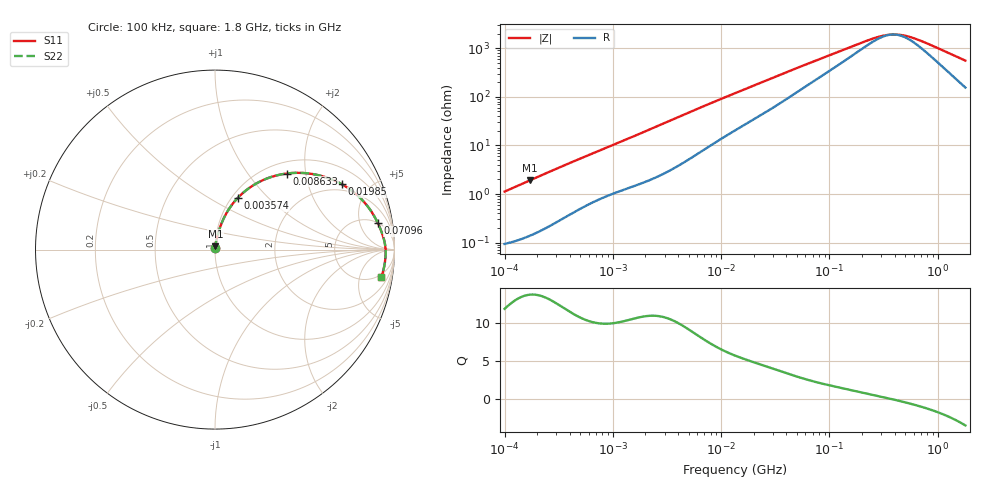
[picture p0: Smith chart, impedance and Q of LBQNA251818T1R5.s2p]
! LBQNA251818T1R5  S-PARAMETER MODEL  ( General Type )
! Model Generated by TAIYO YUDEN Corporation (http://www.ty-top.com)
! Version 1.0
! TAIYO YUDEN Control No. 191025NI43SB-FBB
! Copyright(c) 2019 TAIYO YUDEN CO.,LTD. All Rights Reserved.
! Product Description (link to TY-COMPAS)
! https://ds.yuden.co.jp/TYCOMPAS/or/detail?pn=LBQNA251818T1R5M&u=M
! Products Name : Inductors
! Characteristics :
!  Inductance : 1.5 uH , SRF(min) : 80 MHz , DC Resistance(max) : 0.091 Ohm
!  Rated Current : Saturation :650 mA , Temp Rise : 1100 mA (20 degC)
!  Case Size : 2.5 x 1.8 / 0.098 x 0.071 [mm/inch] , Thickness : 1.8 / 0.071 [mm/inch]
!  (Conditions: Temperature = 25 degC , DC Bias Current/Voltage = 0A / 0V)
! External Node Assignments :
!  1  o---GGG---o  2
! GND o---------o GND
! Frequency Range : 0.1MHz  -  1800MHz  [ 402 STEP ]
# MHz S RI R 50
! Freq[MHz].  S11 Real  S11 Imag  S21 Real  S21 Imag  S12 Real  S12 Imag  S22 Real  S22 Imag
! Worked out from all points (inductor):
!   401 points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, 100 kHz to 1.8 GHz, reference 50 ohm
!   read as one part in series: L = 1.78 uH near 105 kHz
!   highest Q = 13.8 at 171.4 kHz (marker M1), where L = 1.78 uH
!   self-resonance near 382.3 MHz
!   S11 on the Smith chart (normalised r, x): 100 kHz: 1.00, +0.02; 3.574 MHz: 1.07, +0.68; 8.633 MHz: 1.22, +1.57; 19.85 MHz: 1.68, +3.32; 70.96 MHz: 5, +10; 1.8 GHz: 4, -11
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0.1  0.00107 0.0112  0.9989 -0.0112  0.9989 -0.0112  0.00107 0.0112
0.171412  0.00175 0.0191  0.9982 -0.0191  0.9982 -0.0191  0.00175 0.0191
0.516129  0.00813 0.0544  0.9919 -0.0544  0.9919 -0.0544  0.00813 0.0544
1.246616  0.0268 0.1198  0.9732 -0.1198  0.9732 -0.1198  0.0268 0.1198
2.66389  0.0809 0.2308  0.9191 -0.2308  0.9191 -0.2308  0.0809 0.2308
3.574164  0.1272 0.2885  0.8728 -0.2885  0.8728 -0.2885  0.1272 0.2885
5.420303  0.2319 0.3694  0.7681 -0.3694  0.7681 -0.3694  0.2319 0.3694
8.632747  0.3996 0.424  0.6004 -0.424  0.6004 -0.424  0.3996 0.424
13.41641  0.5727 0.4153  0.4273 -0.4153  0.4273 -0.4153  0.5727 0.4153
19.85396  0.7056 0.3648  0.2944 -0.3648  0.2944 -0.3648  0.7056 0.3648
25.99364  0.7768 0.3166  0.2232 -0.3166  0.2232 -0.3166  0.7768 0.3166
34.87589  0.8344 0.2608  0.1656 -0.2608  0.1656 -0.2608  0.8344 0.2608
69.24595  0.9064 0.1496  0.0936 -0.1496  0.0936 -0.1496  0.9064 0.1496
70.9631  0.9079 0.1464  0.0921 -0.1464  0.0921 -0.1464  0.9079 0.1464
121.6389  0.9321 0.0871  0.0679 -0.0871  0.0679 -0.0871  0.9321 0.0871
241.5136  0.9468 0.0317  0.0532 -0.0317  0.0532 -0.0317  0.9468 0.0317
301.0823  0.949 0.0163  0.051 -0.0163  0.051 -0.0163  0.949 0.0163
357.3983  0.9501 0.00459  0.0499 -0.00459  0.0499 -0.00459  0.9501 0.00459
456.5984  0.9508 -0.0123  0.0492 0.0123  0.0492 0.0123  0.9508 -0.0123
597.7978  0.9505 -0.0319  0.0495 0.0319  0.0495 0.0319  0.9505 -0.0319
1076.145  0.9445 -0.0848  0.0555 0.0848  0.0555 0.0848  0.9445 -0.0848
1800  0.9272 -0.1525  0.0728 0.1525  0.0728 0.1525  0.9272 -0.1525
